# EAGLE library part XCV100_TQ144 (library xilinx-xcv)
xcv100_tq144_1532 edit this description Auto generated by make-symbol-device-package-bsdl.ulp Rev. 26 Source: xcv100_tq144_1532.bsd
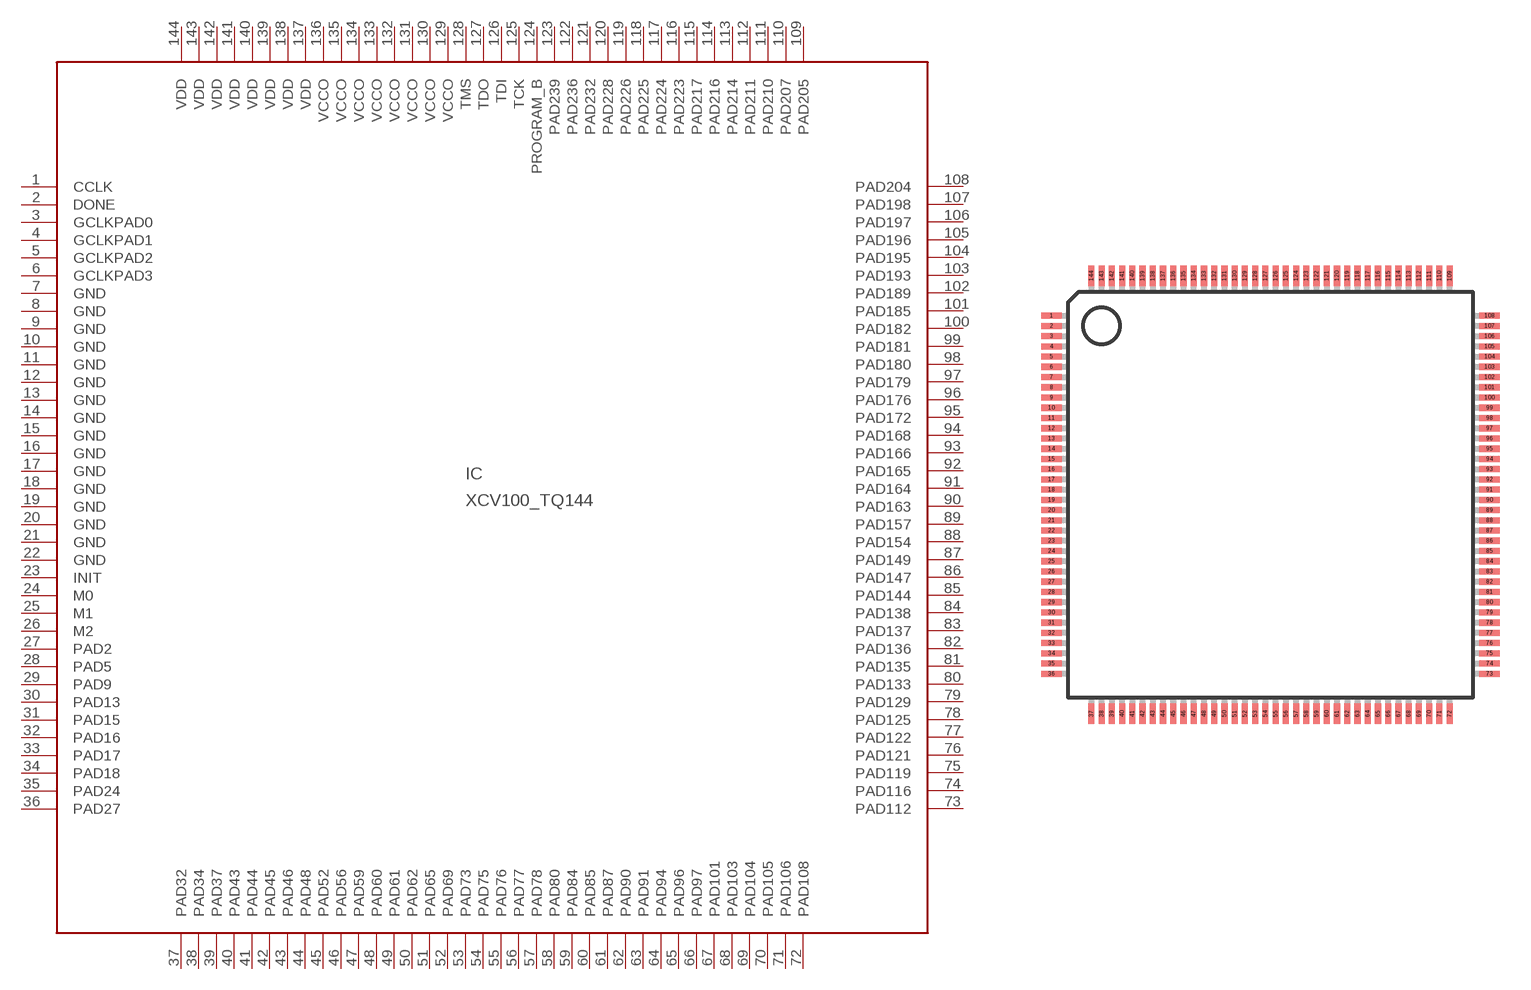
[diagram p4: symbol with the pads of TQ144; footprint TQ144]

Designator prefix IC

## XCV100_TQ144 (OC_FARNELL: unknown; OC_NEWARK: unknown)  [TQ144]
1  CCLK
2  DONE
3  GCLKPAD0  in
4  GCLKPAD1  in
5  GCLKPAD2  in
6  GCLKPAD3  in
7  GND  pwr
8  GND  pwr
9  GND  pwr
10  GND  pwr
11  GND  pwr
12  GND  pwr
13  GND  pwr
14  GND  pwr
15  GND  pwr
16  GND  pwr
17  GND  pwr
18  GND  pwr
19  GND  pwr
20  GND  pwr
21  GND  pwr
22  GND  pwr
23  INIT
24  M0  in
25  M1  in
26  M2  in
27  PAD2
28  PAD5
29  PAD9
30  PAD13
31  PAD15
32  PAD16
33  PAD17
34  PAD18
35  PAD24
36  PAD27
37  PAD32
38  PAD34
39  PAD37
40  PAD43
41  PAD44
42  PAD45
43  PAD46
44  PAD48
45  PAD52
46  PAD56
47  PAD59
48  PAD60
49  PAD61
50  PAD62
51  PAD65
52  PAD69
53  PAD73
54  PAD75
55  PAD76
56  PAD77
57  PAD78
58  PAD80
59  PAD84
60  PAD85
61  PAD87
62  PAD90
63  PAD91
64  PAD94
65  PAD96
66  PAD97
67  PAD101
68  PAD103
69  PAD104
70  PAD105
71  PAD106
72  PAD108
73  PAD112
74  PAD116
75  PAD119
76  PAD121
77  PAD122
78  PAD125
79  PAD129
80  PAD133
81  PAD135
82  PAD136
83  PAD137
84  PAD138
85  PAD144
86  PAD147
87  PAD149
88  PAD154
89  PAD157
90  PAD163
91  PAD164
92  PAD165
93  PAD166
94  PAD168
95  PAD172
96  PAD176
97  PAD179
98  PAD180
99  PAD181
100  PAD182
101  PAD185
102  PAD189
103  PAD193
104  PAD195
105  PAD196
106  PAD197
107  PAD198
108  PAD204
109  PAD205
110  PAD207
111  PAD210
112  PAD211
113  PAD214
114  PAD216
115  PAD217
116  PAD223
117  PAD224
118  PAD225
119  PAD226
120  PAD228
121  PAD232
122  PAD236
123  PAD239
124  PROGRAM_B  in
125  TCK  in
126  TDI  in
127  TDO  out
128  TMS  in
129  VCCO  pwr
130  VCCO  pwr
131  VCCO  pwr
132  VCCO  pwr
133  VCCO  pwr
134  VCCO  pwr
135  VCCO  pwr
136  VCCO  pwr
137  VDD  pwr
138  VDD  pwr
139  VDD  pwr
140  VDD  pwr
141  VDD  pwr
142  VDD  pwr
143  VDD  pwr
144  VDD  pwr

## Footprint TQ144 (pad centres in mm)
TQ144 Auto generated by make-symbol-device-package-bsdl.ulp Rev. 26 Source: xcv100_tq144_1532.bsd; tq144.pdf
smd 1 x 0.3: 1 -10.7,8.75; 2 -10.7,8.25; 3 -10.7,7.75; 4 -10.7,7.25; 5 -10.7,6.75; 6 -10.7,6.25; 7 -10.7,5.75; 8 -10.7,5.25; 9 -10.7,4.75; 10 -10.7,4.25; 11 -10.7,3.75; 12 -10.7,3.25; 13 -10.7,2.75; 14 -10.7,2.25; 15 -10.7,1.75; 16 -10.7,1.25; 17 -10.7,0.75; 18 -10.7,0.25; 19 -10.7,-0.25; 20 -10.7,-0.75; 21 -10.7,-1.25; 22 -10.7,-1.75; 23 -10.7,-2.25; 24 -10.7,-2.75; 25 -10.7,-3.25; 26 -10.7,-3.75; 27 -10.7,-4.25; 28 -10.7,-4.75; 29 -10.7,-5.25; 30 -10.7,-5.75; 31 -10.7,-6.25; 32 -10.7,-6.75; 33 -10.7,-7.25; 34 -10.7,-7.75; 35 -10.7,-8.25; 36 -10.7,-8.75; 73 10.7,-8.75; 74 10.7,-8.25; 75 10.7,-7.75; 76 10.7,-7.25; 77 10.7,-6.75; 78 10.7,-6.25; 79 10.7,-5.75; 80 10.7,-5.25; 81 10.7,-4.75; 82 10.7,-4.25; 83 10.7,-3.75; 84 10.7,-3.25; 85 10.7,-2.75; 86 10.7,-2.25; 87 10.7,-1.75; 88 10.7,-1.25; 89 10.7,-0.75; 90 10.7,-0.25; 91 10.7,0.25; 92 10.7,0.75; 93 10.7,1.25; 94 10.7,1.75; 95 10.7,2.25; 96 10.7,2.75; 97 10.7,3.25; 98 10.7,3.75; 99 10.7,4.25; 100 10.7,4.75; 101 10.7,5.25; 102 10.7,5.75; 103 10.7,6.25; 104 10.7,6.75; 105 10.7,7.25; 106 10.7,7.75; 107 10.7,8.25; 108 10.7,8.75
smd 0.3 x 1: 37 -8.75,-10.7; 38 -8.25,-10.7; 39 -7.75,-10.7; 40 -7.25,-10.7; 41 -6.75,-10.7; 42 -6.25,-10.7; 43 -5.75,-10.7; 44 -5.25,-10.7; 45 -4.75,-10.7; 46 -4.25,-10.7; 47 -3.75,-10.7; 48 -3.25,-10.7; 49 -2.75,-10.7; 50 -2.25,-10.7; 51 -1.75,-10.7; 52 -1.25,-10.7; 53 -0.75,-10.7; 54 -0.25,-10.7; 55 0.25,-10.7; 56 0.75,-10.7; 57 1.25,-10.7; 58 1.75,-10.7; 59 2.25,-10.7; 60 2.75,-10.7; 61 3.25,-10.7; 62 3.75,-10.7; 63 4.25,-10.7; 64 4.75,-10.7; 65 5.25,-10.7; 66 5.75,-10.7; 67 6.25,-10.7; 68 6.75,-10.7; 69 7.25,-10.7; 70 7.75,-10.7; 71 8.25,-10.7; 72 8.75,-10.7; 109 8.75,10.7; 110 8.25,10.7; 111 7.75,10.7; 112 7.25,10.7; 113 6.75,10.7; 114 6.25,10.7; 115 5.75,10.7; 116 5.25,10.7; 117 4.75,10.7; 118 4.25,10.7; 119 3.75,10.7; 120 3.25,10.7; 121 2.75,10.7; 122 2.25,10.7; 123 1.75,10.7; 124 1.25,10.7; 125 0.75,10.7; 126 0.25,10.7; 127 -0.25,10.7; 128 -0.75,10.7; 129 -1.25,10.7; 130 -1.75,10.7; 131 -2.25,10.7; 132 -2.75,10.7; 133 -3.25,10.7; 134 -3.75,10.7; 135 -4.25,10.7; 136 -4.75,10.7; 137 -5.25,10.7; 138 -5.75,10.7; 139 -6.25,10.7; 140 -6.75,10.7; 141 -7.25,10.7; 142 -7.75,10.7; 143 -8.25,10.7; 144 -8.75,10.7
